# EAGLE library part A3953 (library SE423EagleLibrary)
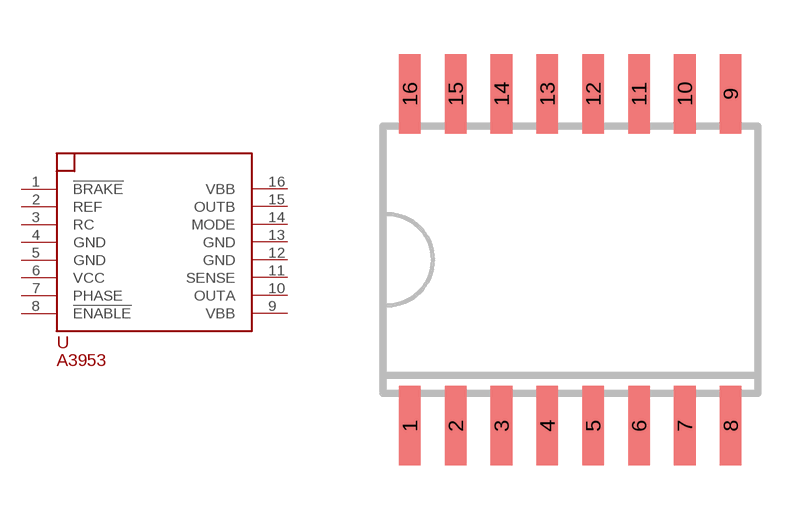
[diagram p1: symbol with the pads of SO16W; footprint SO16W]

Designator prefix U

## A3953  [SO16W]
1  !BRAKE
2  REF
3  RC
4  GND
5  GND
6  VCC
7  PHASE
8  !ENABLE
9  VBB
10  OUTA
11  SENSE
12  GND
13  GND
14  MODE
15  OUTB
16  VBB

## Footprint SO16W (pad centres in mm)
SMALL OUTLINE INTEGRATED CIRCUIT wide body 7.5 mm/JEDEC MS-013AA
smd 0.6 x 2.2: 1 -4.445,-4.6; 2 -3.175,-4.6; 3 -1.905,-4.6; 4 -0.635,-4.6; 5 0.635,-4.6; 6 1.905,-4.6; 7 3.175,-4.6; 8 4.445,-4.6; 9 4.445,4.6; 10 3.175,4.6; 11 1.905,4.6; 12 0.635,4.6; 13 -0.635,4.6; 14 -1.905,4.6; 15 -3.175,4.6; 16 -4.445,4.6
